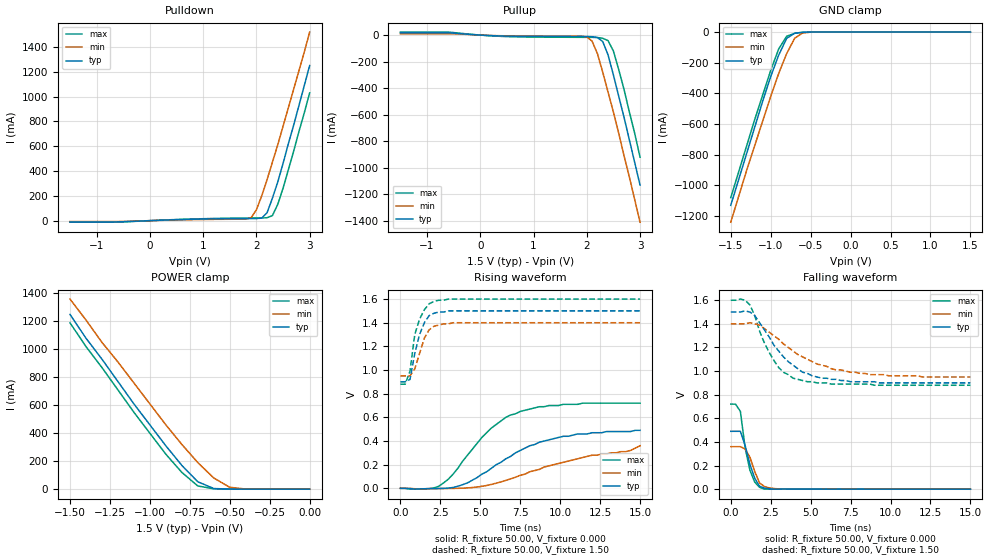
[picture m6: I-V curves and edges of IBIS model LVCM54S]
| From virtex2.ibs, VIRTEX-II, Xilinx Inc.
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|   Model LVCM54S
[Model]   LVCM54S
Model_type   I/O
Polarity   Non-Inverting
Enable   Active-Low
Vinh = 1.05V
Vinl = 0.3V
Vmeas =   0.75V
Cref =  35.00pF
Rref =   1.00M
Vref =  0.000V
C_comp   7.00pF   6.00pF   8.00pF
[Temperature Range]   25.00   100.00   0.000
[Voltage Range]   1.50V   1.40V   1.60V
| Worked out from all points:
|   slope of the pulldown table from 0 to 0.225 V, typ, clamps not added: 59.4 ohm
|   slope of the pullup table from 0 to 0.225 V, typ, clamps not added: 50.4 ohm
|   GND clamp passes 1 mA (typ) near -0.57 V on its own axis
|   POWER clamp passes 1 mA (typ) near -0.52 V on its own axis
|   rising waveform, R_fixture 50.00, V_fixture 0.000: 20-80 % time 3.89ns typ, 5.83ns min, 2.92ns max; typ from 0 V to 0.49 V
|   rising waveform, R_fixture 50.00, V_fixture 1.50: 20-80 % time 704ps typ, 702ps min, 665ps max; typ from 0.9 V to 1.5 V
|   falling waveform, R_fixture 50.00, V_fixture 0.000: 20-80 % time 641ps typ, 618ps min, 566ps max; typ from 0.49 V to 0 V
|   falling waveform, R_fixture 50.00, V_fixture 1.50: 20-80 % time 2.25ns typ, 3.4ns min, 1.51ns max; typ from 1.5 V to 0.9 V
[Pulldown]
| voltage   I(typ)   I(min)   I(max)
-1.5V     -10.77mA   -7.22mA    -12.39mA
-700mV    -10.77mA   -7.22mA    -12.39mA
1.8V      16.48mA    12.48mA    21.06mA
1.9V      16.6mA     23.85mA    21.23mA
2V        16.9mA     87.3mA     21.36mA
2.1V      20.52mA    200mA      21.65mA
2.2V      63.73mA    330mA      23.59mA
2.3V      180mA      470mA      40.3mA
2.4V      310mA      610mA      130mA
2.5V      460mA      760mA      260mA
2.6V      620mA      910mA      410mA
3V        1.25A      1.52A      1.03A
[Pullup]
| voltage   I(typ)   I(min)   I(max)
-1.5V     17.09mA    9.31mA     22.57mA
-600mV    17.09mA    9.31mA     22.57mA
600mV     -8.48mA    -6.17mA    -12.49mA
2V        -11.06mA   -13.11mA   -16.84mA
2.1V      -12.28mA   -46.02mA   -17.04mA
2.2V      -18.12mA   -140mA     -18.41mA
2.3V      -49.07mA   -280mA     -24.56mA
2.4V      -150mA     -430mA     -41.88mA
2.5V      -300mA     -580mA     -120mA
2.7V      -620mA     -910mA     -410mA
2.9V      -960mA     -1.24A     -740mA
3V        -1.13A     -1.41A     -920mA
[GND_clamp]
| voltage   I(typ)   I(min)   I(max)
-1.5V     -1.13A     -1.24A     -1.08A
-1.3V     -790mA     -900mA     -740mA
-1.2V     -620mA     -740mA     -570mA
-1.1V     -450mA     -580mA     -410mA
-1V       -290mA     -420mA     -250mA
-900mV    -150mA     -270mA     -110mA
-800mV    -40.96mA   -140mA     -27.15mA
-700mV    -7.52mA    -40.16mA   -8.06mA
-600mV    -1.38mA    -5.56mA    -1.57mA
-500mV    -120uA     -650uA     -120uA
1.5V      27.96pA    98.69nA    16.96pA
[POWER_clamp]
| voltage   I(typ)   I(min)   I(max)
-1.5V     1.25A      1.36A      1.19A
-1.4V     1.08A      1.21A      1.02A
-1.3V     930mA      1.05A      870mA
-1.2V     770mA      910mA      710mA
-1.1V     610mA      760mA      550mA
-900mV    310mA      460mA      250mA
-800mV    170mA      320mA      120mA
-700mV    52.75mA    190mA      22.81mA
-600mV    4.57mA     79.88mA    2.44mA
-500mV    270uA      13.45mA    250uA
-400mV    16.38uA    820uA      14.46uA
0V        27.96pA    880pA      24.27pA
[Ramp]
| variable   typ   min   max
dV/dt_r   0.29/3.88n   0.19/4.82n   0.43/2.91n
dV/dt_f   0.36/2.25n   0.27/3.31n   0.43/1.55n
R_load = 50.00
[Rising Waveform]
R_fixture = 50.00
V_fixture = 0.000
| time   V(typ)   V(min)   V(max)
0s        0V         0V         0V
2.4ns     -1.64mV    -1.95mV    17.13mV
3.3ns     7.16mV     -640uV     120mV
4.2ns     46.13mV    3.73mV     280mV
5.7ns     170mV      33.06mV    510mV
6.6ns     250mV      67.13mV    600mV
7.5ns     320mV      110mV      650mV
10.2ns    440mV      220mV      710mV
14.1ns    480mV      310mV      720mV
15ns      490mV      360mV      720mV
[Rising Waveform]
R_fixture = 50.00
V_fixture = 1.50
V_fixture_min = 1.40
V_fixture_max = 1.60
| time   V(typ)   V(min)   V(max)
0s        900mV      950mV      880mV
300ps     900mV      950mV      880mV
600ps     920mV      950mV      990mV
900ps     1.14V      1.01V      1.3V
1.2ns     1.3V       1.14V      1.43V
1.5ns     1.4V       1.27V      1.51V
1.8ns     1.46V      1.34V      1.56V
2.1ns     1.48V      1.37V      1.58V
3.3ns     1.5V       1.4V       1.6V
15ns      1.5V       1.4V       1.6V
[Falling Waveform]
R_fixture = 50.00
V_fixture = 0.000
| time   V(typ)   V(min)   V(max)
0s        490mV      360mV      720mV
300ps     490mV      360mV      720mV
600ps     490mV      360mV      660mV
900ps     370mV      340mV      350mV
1.2ns     210mV      270mV      160mV
1.5ns     92.58mV    150mV      59.68mV
1.8ns     24.84mV    52.99mV    16.15mV
2.1ns     9.86mV     23.18mV    240uV
3.3ns     610uV      590uV      560uV
15ns      6.45uV     27.1uV     33.55uV
[Falling Waveform]
R_fixture = 50.00
V_fixture = 1.50
V_fixture_min = 1.40
V_fixture_max = 1.60
| time   V(typ)   V(min)   V(max)
0s        1.5V       1.4V       1.6V
600ps     1.5V       1.4V       1.61V
1.2ns     1.5V       1.41V      1.56V
2.1ns     1.35V      1.36V      1.24V
2.7ns     1.22V      1.3V       1.09V
3.3ns     1.12V      1.23V      990mV
3.9ns     1.05V      1.17V      940mV
5.1ns     960mV      1.08V      910mV
7.5ns     910mV      990mV      890mV
15ns      900mV      950mV      880mV
